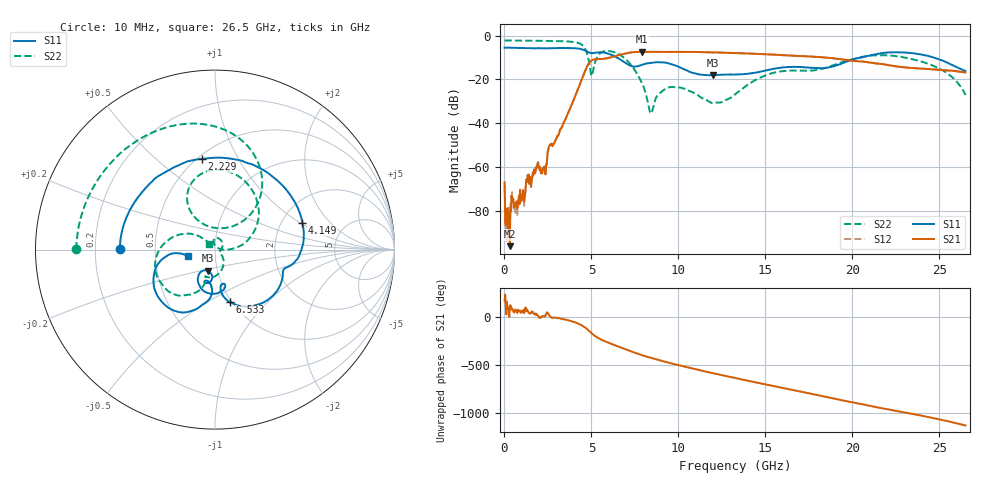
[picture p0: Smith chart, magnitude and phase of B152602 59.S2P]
!  2-Port S-parameters saved by WinCal
! VAR MeasName=S-Parameters (CALIBRATED_DATA) read from VNA (N5242A)
! VAR MeasDate=2016-1-5 16:34:18
! VAR NAME=B152602 59
! VAR FILENAME=B152602 59.S2P
! VAR DATE=2016-1-5 16:34:18
! VAR PHYS_PORTS=1,2
# Hz S DB R 50
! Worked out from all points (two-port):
!   801 points, 10 MHz to 26.5 GHz, reference 50 ohm
!   highest |S21| = -7.42 dB at 7.924 GHz (marker M1); lowest = -96.2 dB at 308 MHz (marker M2)
!   |S21| within 3 dB of the highest: 5.861 GHz to 18.93 GHz (13.07 GHz wide, 105 % of centre)
!   lowest |S11| = -18.1 dB at 12 GHz (marker M3), VSWR 1.28, Z = 44.8 - j10.6 ohm
!   |S11| at or under -10 dB: 6.45 GHz to 20.51 GHz (14.06 GHz wide, 104 % of centre); 24.66 GHz to end of sweep
!   |S22| runs from -35.6 to -2.2 dB; largest |S21 - S12| = 0.0029
!   S11 on the Smith chart (normalised r, x): 10 MHz: 0.31, +0.00; 2.229 GHz: 0.52, +0.72; 4.149 GHz: 2.59, +1.05; 6.533 GHz: 0.98, -0.63; 26.5 GHz: 0.74, -0.06
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1e7  -5.53 179.6  -67.03 175.2  -68.69 -32.3  -2.23 179.8
3.080125e8  -5.54 168.5  -96.20 86.0  -89.52 140.2  -2.25 175.2
1.0696e9  -5.73 141.0  -70.60 51.6  -71.21 56.3  -2.30 163.4
1.831188e9  -5.82 113.5  -59.91 28.8  -60.38 27.9  -2.37 151.1
2.228538e9  -5.83 98.3  -60.48 12.1  -60.58 12.9  -2.42 144.2
4.149062e9  -5.86 17.1  -26.02 -58.1  -26.04 -57.9  -3.17 92.6
4.447075e9  -6.24 2.1  -19.91 -83.5  -19.90 -83.3  -4.18 74.7
5.009988e9  -8.01 -16.4  -11.37 -165.7  -11.37 -165.5  -18.42 81.1
5.5729e9  -7.66 -35.4  -10.72 127.1  -10.72 127.2  -7.70 105.2
6.533162e9  -10.31 -74.1  -9.03 56.7  -9.02 56.8  -8.31 56.0
7.923888e9  -13.28 -74.9  -7.42 -35.1  -7.42 -35.0  -22.01 0.5
8.420575e9  -12.48 -83.4  -7.46 -62.2  -7.45 -62.3  -35.61 53.6
8.851038e9  -12.18 -93.5  -7.47 -84.3  -7.43 -84.4  -26.97 98.6
1.050666e10  -16.04 -123.1  -7.46 -160.5  -7.44 -160.3  -24.74 49.7
1.199672e10  -18.14 -109.5  -7.70 137.5  -7.68 137.3  -30.91 -16.7
1.3255e10  -17.81 -104.2  -7.99 87.8  -7.97 87.8  -26.89 -38.9
1.540731e10  -15.29 -96.7  -8.70 6.1  -8.65 6.1  -17.16 -83.6
1.769208e10  -14.74 -108.0  -9.63 -78.6  -9.59 -78.4  -15.96 -109.5
1.974505e10  -11.64 -94.9  -11.30 -156.2  -11.24 -156.2  -11.35 -115.9
2.209604e10  -7.71 -125.5  -13.58 119.0  -13.49 118.6  -9.07 -160.5
2.500994e10  -10.93 -171.3  -15.64 16.8  -15.64 16.7  -15.14 149.5
2.65e10  -16.15 -165.7  -16.86 -46.4  -16.85 -46.4  -27.18 134.9
